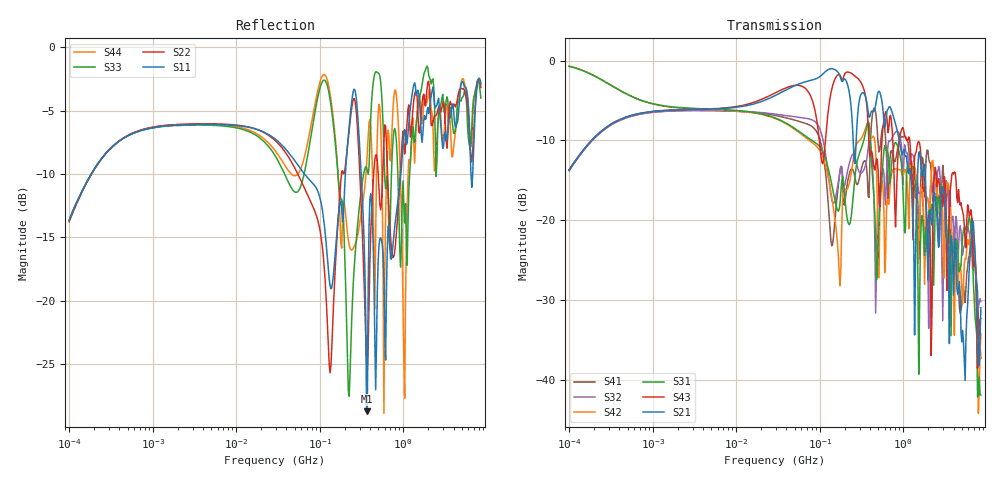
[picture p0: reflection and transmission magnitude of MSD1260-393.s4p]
# MHz S MA R 50
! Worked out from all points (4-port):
!   498 points, 100 kHz to 8.5 GHz, reference 50 ohm
!   strongest paths, dB at 100 kHz, 1.698 MHz, 29.49 MHz, 500.7 MHz, 8.5 GHz:
!     S21: -13.7, -6.2, -4.4, -3.9, -30.9
!     S43: -13.7, -6.2, -4.0, -13.8, -32.3
!     S31: -0.7, -5.8, -7.2, -22.4, -41.9
!     S42: -0.7, -5.8, -7.3, -27.1, -34.2
!     S32: -13.8, -6.3, -6.7, -17.2, -30.2
!     S41: -13.8, -6.3, -6.9, -10.4, -37.3
!   lowest |S11| = -28.7 dB at 363.7 MHz (marker M1), VSWR 1.08, Z = 48.8 - j3.39 ohm
!   |S11| at or under -10 dB: 65.91 MHz to 203 MHz (137.1 MHz wide, 102 % of centre); 313.6 MHz to 935 MHz (621.4 MHz wide, 99.5 % of centre); 6.469 GHz to 6.784 GHz (314.8 MHz wide, 4.75 % of centre)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
0.1  0.2084 63.6  0.2073 63.8  0.9206 -11.8  0.2047 -116.5
     0.2073 63.8  0.2048 63.8  0.205 -116.3  0.9226 -11.7
     0.9206 -11.8  0.205 -116.3  0.2074 63.7  0.2066 63.7
     0.2047 -116.5  0.9226 -11.7  0.2066 63.7  0.2076 63.8
133.1311  0.1144 -28.8  0.887 -24.8  0.1882 99.2  0.08652 0.6
          0.887 -24.8  0.05194 -12.9  0.157 -6.4  0.1611 106.5
          0.1882 99.2  0.157 -6.4  0.6232 -64.9  0.5858 14.8
          0.08652 0.6  0.1611 106.5  0.5858 14.8  0.6554 -57.5
258.1735  0.6837 -40.4  0.2378 -67.6  0.1646 63.9  0.1968 15.0
          0.2378 -67.6  0.6277 -46.6  0.2577 -6.3  0.2602 68.9
          0.1646 63.9  0.2577 -6.3  0.1337 48.6  0.8077 -56.3
          0.1968 15.0  0.2602 68.9  0.8077 -56.3  0.1636 -30.9
363.6528  0.03658 -108.2  0.5589 -68.9  0.3803 -12.2  0.2157 -1.1
          0.5589 -68.9  0.0565 -174.4  0.2375 -17.0  0.3948 -4.0
          0.3803 -12.2  0.2375 -17.0  0.3363 6.0  0.54 -111.6
          0.2157 -1.1  0.3948 -4.0  0.54 -111.6  0.342 -13.9
1970.81  0.5794 -157.6  0.04238 99.9  0.0706 -176.0  0.275 156.0
         0.04238 99.9  0.7282 -165.2  0.05161 119.2  0.1382 170.8
         0.0706 -176.0  0.05161 119.2  0.8291 -169.5  0.08292 126.3
         0.275 156.0  0.1382 170.8  0.08292 126.3  0.628 -158.9
3409.455  0.4727 47.4  0.07046 -71.7  0.06311 13.9  0.169 -18.0
          0.07046 -71.7  0.44 36.8  0.156 11.4  0.1721 7.8
          0.06311 13.9  0.156 11.4  0.6184 8.8  0.04775 75.6
          0.169 -18.0  0.1721 7.8  0.04775 75.6  0.5265 29.8
8500  0.7173 -55.2  0.02836 -46.3  0.008064 -30.0  0.01365 -126.1
      0.02836 -46.3  0.6943 -57.3  0.031 -134.4  0.01959 -54.3
      0.008064 -30.0  0.031 -134.4  0.63 -55.3  0.02432 -36.8
      0.01365 -126.1  0.01959 -54.3  0.02432 -36.8  0.7253 -56.4
